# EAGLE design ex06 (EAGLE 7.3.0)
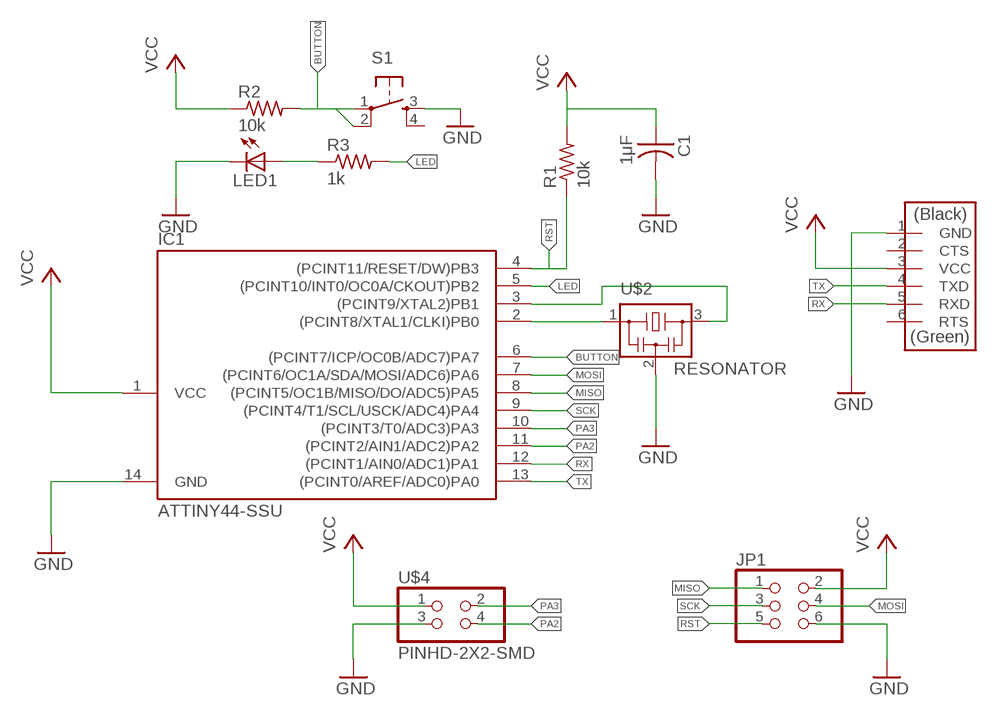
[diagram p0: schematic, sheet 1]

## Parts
C1  1μF  CAP-US1206FAB  [C1206FAB]
IC1  ATTINY44-SSU  [SOIC14]
JP1  PINHD-2X3-SMD  [2X03SMD]
LED1  LEDCHIP-LED0805  [CHIP-LED0805]
R1  10k  RES-US1206FAB  [R1206FAB]
R2  10k  RES-US1206FAB  [R1206FAB]
R3  1k  RES-US1206FAB  [R1206FAB]
S1  6MM_SWITCH6MM_SWITCH  [6MM_SWITCH]
U$2  RESONATOR  [EFOBM]
U$3  FTDI-SMD-HEADER  [1X06SMD]
U$4  PINHD-2X2-SMD  [2X02SMD]

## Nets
BUTTON: IC1.6((PCINT7/ICP/OC0B/ADC7)PA7) R2.2 S1.1(P) S1.2(P1)
GND: C1.2 IC1.14(GND) JP1.6 LED1.C S1.3(S) U$2.2 U$3.1(GND) U$4.3
LED: IC1.5((PCINT10/INT0/OC0A/CKOUT)PB2) R3.2
MISO: IC1.8((PCINT5/OC1B/MISO/DO/ADC5)PA5) JP1.1
MOSI: IC1.7((PCINT6/OC1A/SDA/MOSI/ADC6)PA6) JP1.4
N$2: IC1.2((PCINT8/XTAL1/CLKI)PB0) U$2.1
N$3: IC1.3((PCINT9/XTAL2)PB1) U$2.3
N$6: LED1.A R3.1
PA2: IC1.11((PCINT2/AIN1/ADC2)PA2) U$4.4
PA3: IC1.10((PCINT3/T0/ADC3)PA3) U$4.2
RST: IC1.4((PCINT11/RESET/DW)PB3) JP1.5 R1.1
RX: IC1.12((PCINT1/AIN0/ADC1)PA1) U$3.5(RXD)
SCK: IC1.9((PCINT4/T1/SCL/USCK/ADC4)PA4) JP1.3
TX: IC1.13((PCINT0/AREF/ADC0)PA0) U$3.4(TXD)
VCC: C1.1 IC1.1(VCC) JP1.2 R1.2 R2.1 U$3.3(VCC) U$4.1
Unconnected: S1.4(S1) U$3.2(CTS) U$3.6(RTS)

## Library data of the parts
C1 = fab:CAP-US
IC1 = fab:ATTINY44
JP1 = fab:PINHD-2X3-SMD: PIN HEADER
LED1 = led:LED: LED
R1-R3 = fab:RES-US: Resistor (US Symbol)
S1 = fab:6MM_SWITCH: OMRON SWITCH
U$2 = fab:RESONATOR
U$3 = fab:FTDI-SMD-HEADER
U$4 = fab:PINHD-2X2-SMD

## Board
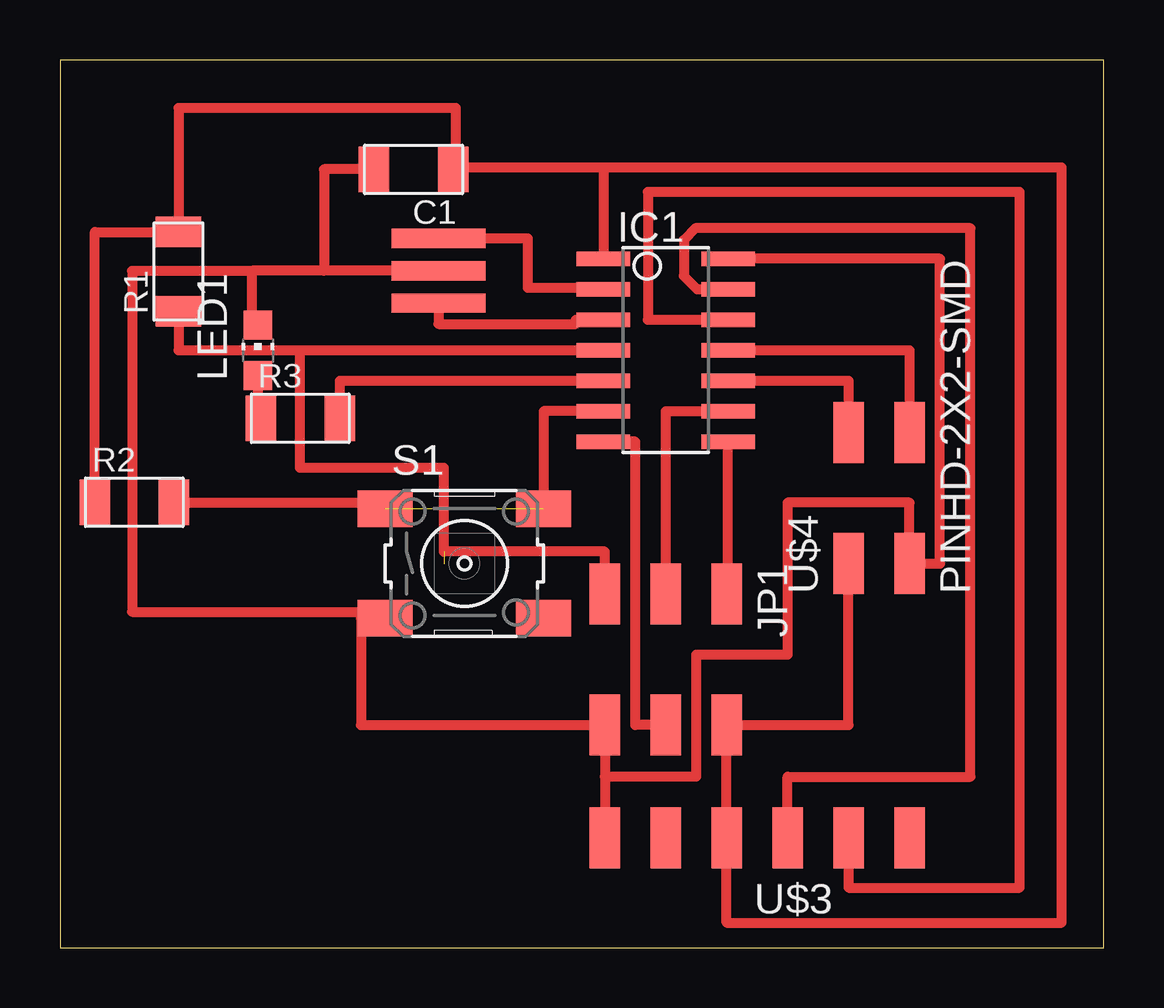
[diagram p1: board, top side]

Size 43.5 x 37 mm. Coordinates in mm from the lower left corner, seen from the top.
Outline: 0,0 43.5,0 43.5,37 0,37 0,0
Copper layers (1*16): Top 0.035mm / dielectric 1.5mm / Bottom 0.035mm
Design rules "default": minimum track width 10mil, minimum drill 24mil, track to track 8mil, track to pad 8mil, pad to pad 8mil, via to via 8mil, smd to smd 8mil, copper to edge 40mil, drill to drill 8mil, minimum pad ring 10mil, minimum via ring 8mil, stop-mask expansion 4mil, vias tented up to drill 0mil, thermal gap 10mil

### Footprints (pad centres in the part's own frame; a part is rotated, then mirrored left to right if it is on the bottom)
C1206FAB = smd 1.27 x 1.905: 1 -1.651,0; 2 1.651,0
SOIC14 = smd 0.61 x 2.21: 1 -3.81,-2.603; 2 -2.54,-2.603; 3 -1.27,-2.603; 4 0,-2.603; 5 1.27,-2.603; 6 2.54,-2.603; 7 3.81,-2.603; 8 3.81,2.603; 9 2.54,2.603; 10 1.27,2.603; 11 0,2.603; 12 -1.27,2.603; 13 -2.54,2.603; 14 -3.81,2.603
2X03SMD = smd 2.54 x 1.27: 1 -2.54,2.54; 2 2.92,2.54; 3 -2.54,0; 4 2.92,0; 5 -2.54,-2.54; 6 2.92,-2.54
CHIP-LED0805 = smd 1.2 x 1.2: A 0,-1.05; C 0,1.05
R1206FAB = smd 1.27 x 1.905: 1 -1.651,0; 2 1.651,0
6MM_SWITCH = smd 2.286 x 1.524: 1 -3.302,2.286; 2 3.302,2.286; 3 -3.302,-2.286; 4 3.302,-2.286
EFOBM = smd 0.8 x 3.9: 1 -1.35,0; 2 0,0; 3 1.35,0
1X06SMD = smd 2.54 x 1.27: 1 0,6.35; 2 0,3.81; 3 0,1.27; 4 0,-1.27; 5 0,-3.81; 6 0,-6.35
2X02SMD = smd 2.54 x 1.27: 1 -2.54,1.27; 2 2.92,1.27; 3 -2.54,-1.27; 4 2.92,-1.27

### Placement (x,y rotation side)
C1  14.74,32.44 180 top
IC1  25.25,24.9 270 top
JP1  25.25,12.2 270 top
LED1  8.25,24.9 0 top
R1  4.94,28.18 90 top
R2  3.1,18.56 0 top
R3  10.02,22.06 0 top
S1  16.86,16.01 0 top
U$2  15.78,28.21 270 top
U$3  29.06,4.58 90 top
U$4  34.14,18.55 90 top

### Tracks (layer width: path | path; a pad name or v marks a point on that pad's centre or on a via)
BUTTON  (1 unrouted)
  Top 0.406: S1.1 13.56,18.56 R2.2 | IC1.6 20.16,22.36 S1.2
GND
  Top 0.406: S1.3 12.55,13.72 | 22.71,7.12 JP1.6 12.55,9.28 12.55,13.72 | 22.71,7.12 U$3.1 | IC1.14 36.68,28.71 36.68,16.01 U$4.3 35.41,18.55 30.33,18.55 30.33,12.2 26.52,12.2 26.52,7.12 22.71,7.12 | 8,28.21 3,28.21 3,14 12.55,14 12.55,13.72 | U$2.2 11,28.21 | 11,28.21 8,28.21 | LED1.C 8,26.45 8,28.21 | C1.2 11,32.44 11,28.21
LED
  Top 0.406: R3.2 11.67,23.63 IC1.5
MISO
  Top 0.406: JP1.1 27.85,14.74 IC1.8
MOSI
  Top 0.406: JP1.4 23.98,9.28 23.98,21.09 IC1.7
N$2
  Top 0.406: IC1.2 22.65,27.5 19.5,27.5 19.5,29.56 U$2.1
N$3
  Top 0.406: U$2.3 15.78,26 21.5,26 21.5,26.17 IC1.3
N$6
  Top 0.406: R3.1 8.25,22.06 LED1.A
PA2
  Top 0.406: IC1.11 35.41,24.9 U$4.4
PA3
  Top 0.406: IC1.10 32.87,23.63 U$4.2
RST  (1 unrouted)
  Top 0.406: JP1.5 22.71,16.51 16,16.51 16,20 10,20 10,24.9 | 10,24.9 IC1.4 | R1.1 4.94,24.9 10,24.9
RX
  Top 0.406: U$3.5 32.87,2.5 40,2.5 40,31.5 24.5,31.5 24.5,26.17 IC1.12
SCK
  Top 0.406: JP1.3 25.25,22.36 IC1.9
TX
  Top 0.406: U$3.4 30.33,7.12 37.95,7.12 37.95,29.98 26.48,29.98 26,29.5 26,28 26.56,27.44 IC1.13
VCC
  Top 0.406: U$4.1 32.87,9.28 JP1.2 U$3.3 27.79,1.04 41.76,1.04 41.76,32.52 22.65,32.52 | 22.65,32.52 IC1.1 | 22.65,32.52 16.39,32.52 C1.1 16.5,32.44 16.5,35 4.94,35 R1.2 1.45,29.83 R2.1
